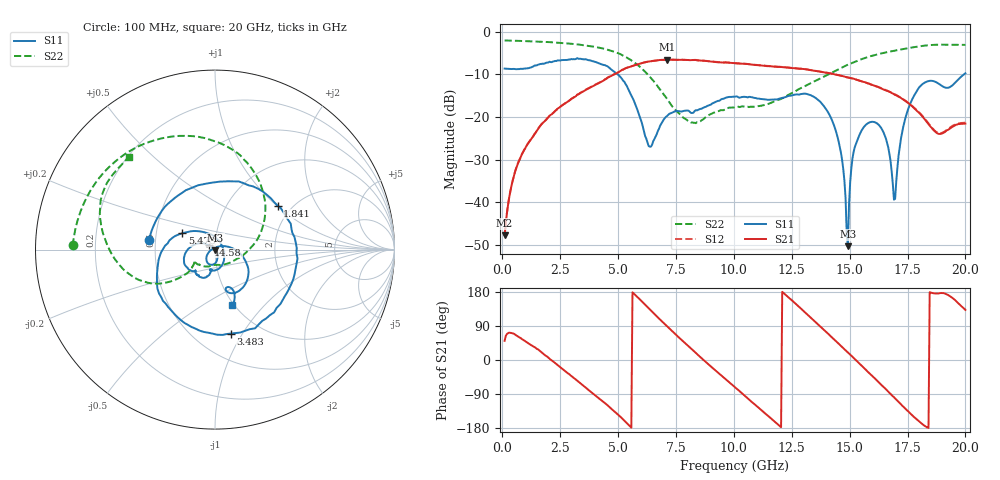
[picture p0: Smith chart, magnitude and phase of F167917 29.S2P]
!  2-Port S-parameters saved by WinCal
! VAR MeasName=S-Parameters (CALIBRATED_DATA) read from VNA (N5242A)
! VAR MeasDate=2016-11-22 9:01:09
! VAR NAME=F167917 29
! VAR FILENAME=F167917 29.S2P
! VAR DATE=2016-11-22 9:01:09
! VAR PHYS_PORTS=1,2
# Hz S DB R 50
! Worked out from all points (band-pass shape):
!   401 points, 100 MHz to 20 GHz, reference 50 ohm
!   highest |S21| = -6.54 dB at 7.115 GHz (marker M1); lowest = -47.7 dB at 100 MHz (marker M2)
!   |S21| within 3 dB of the highest: 5.002 GHz to 13.91 GHz (8.913 GHz wide, 94.2 % of centre)
!   lowest |S11| = -50.3 dB at 14.93 GHz (marker M3), VSWR 1.01, Z = 50.2 - j0.181 ohm
!   |S11| at or under -10 dB: 4.99 GHz to 19.94 GHz (14.94 GHz wide, 120 % of centre)
!   |S22| runs from -21.4 to -2.0 dB; largest |S21 - S12| = 0.0043
!   S11 on the Smith chart (normalised r, x): 100 MHz: 0.46, +0.06; 1.841 GHz: 1.69, +1.01; 3.483 GHz: 0.74, -0.89; 5.473 GHz: 0.68, +0.13; 14.58 GHz: 0.93, +0.05; 20 GHz: 0.98, -0.68
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1e8  -8.63 171.5  -47.75 50.5  -47.68 51.3  -2.03 178.3
6.4725e8  -8.76 127.6  -31.31 63.4  -31.29 63.4  -2.11 169.6
1.84125e9  -7.41 35.0  -20.90 12.9  -20.90 12.7  -2.36 150.6
3.43325e9  -6.40 -76.3  -14.19 -64.6  -14.13 -64.4  -3.08 121.0
3.483e9  -6.44 -79.3  -14.04 -67.0  -13.97 -66.9  -3.11 119.9
5.473e9  -13.84 153.3  -8.25 -172.5  -8.23 -172.9  -6.35 62.7
6.31875e9  -26.79 40.2  -6.99 136.5  -6.99 136.4  -10.23 28.4
6.7665e9  -22.75 -46.2  -6.63 109.6  -6.64 109.6  -13.22 7.7
7.11475e9  -19.76 -73.6  -6.54 88.9  -6.55 89.0  -15.74 -9.7
8.5575e9  -18.09 -101.1  -6.73 7.4  -6.71 7.5  -21.00 -100.5
1.005e10  -15.23 -119.0  -7.38 -71.9  -7.37 -71.9  -17.69 -145.8
1.1841e10  -15.88 -133.4  -8.23 -166.7  -8.19 -166.6  -16.13 -143.0
1.338325e10  -15.06 -166.6  -9.02 108.0  -9.02 108.2  -11.88 -141.6
1.457725e10  -27.05 141.9  -10.23 40.0  -10.23 40.2  -8.64 -149.2
1.49255e10  -50.31 -36.3  -10.73 20.0  -10.70 20.2  -7.71 -153.1
1.517425e10  -28.13 -65.5  -11.01 5.2  -11.03 5.5  -7.15 -156.4
1.5622e10  -22.28 -89.5  -11.78 -21.0  -11.79 -20.8  -6.22 -162.8
1.67165e10  -28.57 -157.3  -14.04 -86.3  -14.06 -85.8  -4.66 -179.3
1.696525e10  -39.19 89.0  -14.83 -101.5  -14.70 -100.8  -4.40 177.2
1.736325e10  -21.24 7.8  -16.08 -125.9  -16.00 -125.0  -3.99 171.6
1.79105e10  -13.82 -27.0  -18.57 -157.2  -18.43 -156.6  -3.50 163.4
2e10  -9.74 -72.8  -21.55 132.1  -21.33 132.3  -3.06 133.0
